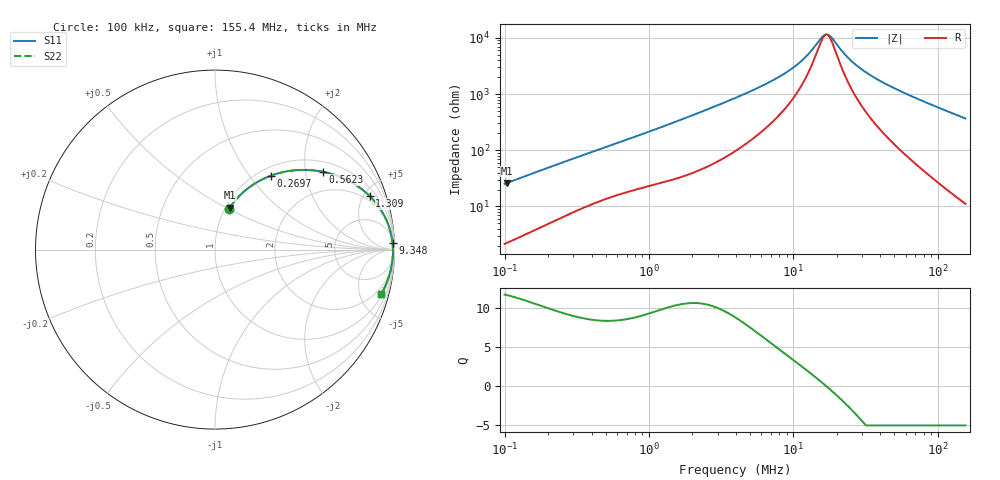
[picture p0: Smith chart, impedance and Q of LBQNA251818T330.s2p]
! LBQNA251818T330  S-PARAMETER MODEL  ( General Type )
! Model Generated by TAIYO YUDEN Corporation (http://www.ty-top.com)
! Version 1.0
! TAIYO YUDEN Control No. 191025NI43SB-FBB
! Copyright(c) 2019 TAIYO YUDEN CO.,LTD. All Rights Reserved.
! Product Description (link to TY-COMPAS)
! https://ds.yuden.co.jp/TYCOMPAS/or/detail?pn=LBQNA251818T330K&u=M
! Products Name : Inductors
! Characteristics :
!  Inductance : 33 uH , SRF(min) : 15 MHz , DC Resistance(max) : 0.91 Ohm
!  Rated Current : Saturation :130 mA , Temp Rise : 320 mA (20 degC)
!  Case Size : 2.5 x 1.8 / 0.098 x 0.071 [mm/inch] , Thickness : 1.8 / 0.071 [mm/inch]
!  (Conditions: Temperature = 25 degC , DC Bias Current/Voltage = 0A / 0V)
! External Node Assignments :
!  1  o---GGG---o  2
! GND o---------o GND
! Frequency Range : 0.1MHz  -  155.401204MHz  [ 402 STEP ]
# MHz S RI R 50
! Freq[MHz].  S11 Real  S11 Imag  S21 Real  S21 Imag  S12 Real  S12 Imag  S22 Real  S22 Imag
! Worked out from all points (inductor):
!   401 points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, 100 kHz to 155.4 MHz, reference 50 ohm
!   read as one part in series: L = 39.6 uH near 103.7 kHz
!   highest Q = 11.6 at 103.7 kHz (marker M1), where L = 40 uH
!   self-resonance near 16.83 MHz
!   S11 on the Smith chart (normalised r, x): 100 kHz: 1.04, +0.50; 269.7 kHz: 1.14, +1.28; 562.3 kHz: 1.30, +2.51; 1.309 MHz: 1.55, +5.51; 9.348 MHz: 15, +51; 155.4 MHz: 1.22, -7.35
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0.1  0.077 0.2272  0.923 -0.2272  0.923 -0.2272  0.077 0.2272
0.103743  0.0816 0.234  0.9184 -0.234  0.9184 -0.234  0.0816 0.234
0.167264  0.1679 0.3289  0.8321 -0.3289  0.8321 -0.3289  0.1679 0.3289
0.269679  0.3127 0.4123  0.6873 -0.4123  0.6873 -0.4123  0.3127 0.4123
0.342427  0.4036 0.4365  0.5964 -0.4365  0.5964 -0.4365  0.4036 0.4365
0.562331  0.6025 0.4332  0.3975 -0.4332  0.3975 -0.4332  0.6025 0.4332
1.172566  0.8373 0.3211  0.1627 -0.3211  0.1627 -0.3211  0.8373 0.3211
1.309209  0.8615 0.2988  0.1385 -0.2988  0.1385 -0.2988  0.8615 0.2988
2.149969  0.9359 0.2023  0.0641 -0.2023  0.0641 -0.2023  0.9359 0.2023
3.942096  0.9739 0.1125  0.0261 -0.1125  0.0261 -0.1125  0.9739 0.1125
6.593697  0.9855 0.0617  0.0145 -0.0617  0.0145 -0.0617  0.9855 0.0617
9.348094  0.989 0.0361  0.011 -0.0361  0.011 -0.0361  0.989 0.0361
11.44163  0.9902 0.0232  0.00982 -0.0232  0.00982 -0.0232  0.9902 0.0232
13.49882  0.9909 0.0132  0.00914 -0.0132  0.00914 -0.0132  0.9909 0.0132
15.92588  0.9913 0.00354  0.0087 -0.00354  0.0087 -0.00354  0.9913 0.00354
17.45809  0.9914 -0.0018  0.00856 0.0018  0.00856 0.0018  0.9914 -0.0018
22.99727  0.9914 -0.0182  0.00857 0.0182  0.00857 0.0182  0.9914 -0.0182
27.13214  0.9911 -0.0287  0.00892 0.0287  0.00892 0.0287  0.9911 -0.0287
34.45135  0.99 -0.0453  0.01 0.0453  0.01 0.0453  0.99 -0.0453
46.22367  0.9873 -0.0693  0.0127 0.0693  0.0127 0.0693  0.9873 -0.0693
80.20907  0.9745 -0.1312  0.0255 0.1312  0.0255 0.1312  0.9745 -0.1312
155.4012  0.9246 -0.2494  0.0754 0.2494  0.0754 0.2494  0.9246 -0.2494
